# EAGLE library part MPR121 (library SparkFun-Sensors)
NXP MPR121 Proximity Capacitive Touch Sensor Controller The MPR121 is a capacitive touch sensor controller driven by an I2C interface. The chip can control up to twelve individual electrodes, as well as a simulated thirteenth electrode. The MPR121 also features eight LED driving pins. When these pins are not configured as electrodes, they may be used to drive LEDs. Datasheet SparkFun Products Capacitive Touch Sensor Controller - MPR121QR2 (COM-09604) SparkFun Capacitive Touch Sensor Breakout - MPR121 (SEN-09695) SparkFun Touch Shield (DEV-12013) SparkFun Capacitive Touch Keypad - MPR121 (SEN-12017)
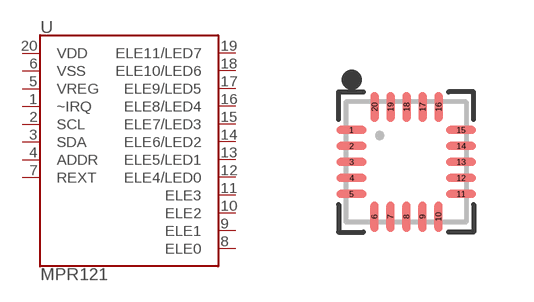
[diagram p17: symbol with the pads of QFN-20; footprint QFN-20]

Designator prefix U

## MPR121 (PROD_ID: IC-09490; SF_ID: COM-09604)  [QFN-20]
1  ~IRQ
2  SCL
3  SDA
4  ADDR
5  VREG
6  VSS
7  REXT
8  ELE0
9  ELE1
10  ELE2
11  ELE3
12  ELE4/LED0
13  ELE5/LED1
14  ELE6/LED2
15  ELE7/LED3
16  ELE8/LED4
17  ELE9/LED5
18  ELE10/LED6
19  ELE11/LED7
20  VDD

## Footprint QFN-20 (pad centres in mm)
20-Pin Quad Flat No-Lead (QFN) (3 x 3 mm) Datasheet Specifications: Pin Count: 20 Dimensions: 3.0 x 3.0 x 0.65 mm Pitch: 0.4 mm Devices Using: MPR121
smd 0.75 x 0.195: 1 -1.367,0.8; 2 -1.367,0.4; 3 -1.367,0; 4 -1.367,-0.4; 5 -1.367,-0.8; 11 1.375,-0.8; 12 1.375,-0.4; 13 1.375,0; 14 1.375,0.4; 15 1.375,0.8
smd 0.195 x 0.75: 6 -0.795,-1.372; 7 -0.395,-1.372; 8 0.005,-1.372; 9 0.405,-1.372; 10 0.805,-1.372; 16 0.81,1.372; 17 0.41,1.372; 18 0.01,1.372; 19 -0.39,1.372; 20 -0.79,1.372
